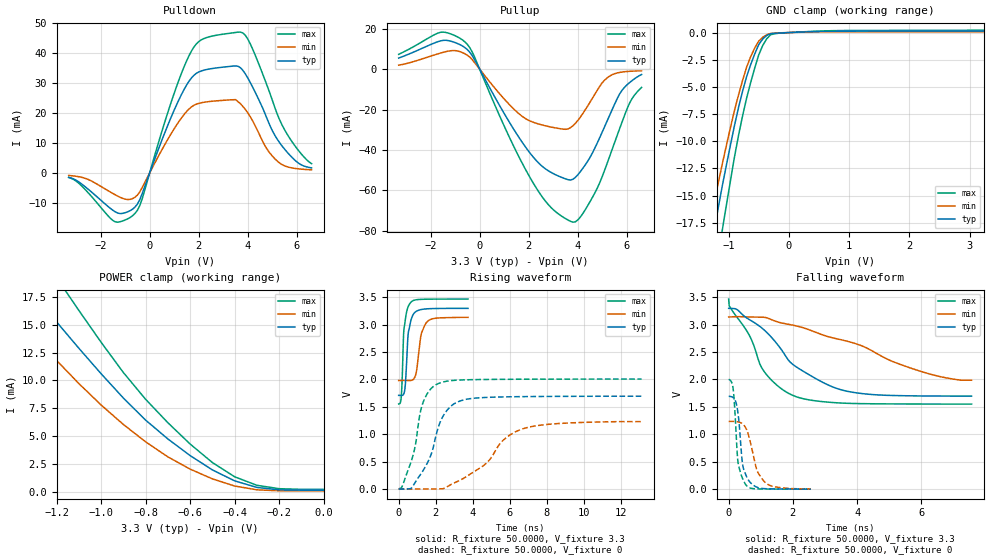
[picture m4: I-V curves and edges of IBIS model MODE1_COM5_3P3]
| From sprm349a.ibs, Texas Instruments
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|MODE4_IND5_3P3BUFFER IN NORMAL MODE WITH INDTEMP AT PLUS OR MINUS 5PERCENT
| VDDS
|COM AND INDE ARE TWO DIFFERENT TEMP MODES.
|COM IS 25,0,105(NOM,STRONG,WEAK)
|IND IS 25,-40,125(NOM,STRONG,WEAK)
|   Model Cell MODE1_COM5_3P3
|MODE1_COM5_3P3
[Model]   MODE1_COM5_3P3
Model_type   I/O
Polarity   Non-Inverting
Enable   Active-Low
Vinl =  0.8V
Vinh =  2V
Cref =  15.0000pF
Rref =  100.0000M
Vref =  0V
Vmeas =  1.65
C_comp   1.505368p   1.470769p   1.543249p
[Model Spec]
Vinl   0.8V   0.8V   0.8V
Vinh   2V   2V   2V
[Temperature Range]   25   105   0
[Voltage Range]   3.3   3.14   3.47
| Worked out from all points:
|   slope of the pulldown table from 0 to 0.495 V, typ, clamps not added: 45.6 ohm
|   slope of the pullup table from 0 to 0.495 V, typ, clamps not added: 44.5 ohm
|   GND clamp passes 1 mA (typ) near -0.49 V on its own axis
|   POWER clamp passes 1 mA (typ) near -0.40 V on its own axis
|   rising waveform, R_fixture 50.0000, V_fixture 3.3: 20-80 % time 216ps typ, 314ps min, 177ps max; typ from 1.71 V to 3.3 V
|   rising waveform, R_fixture 50.0000, V_fixture 0: 20-80 % time 1.12ns typ, 2.25ns min, 778ps max; typ from 0 V to 1.69 V
|   falling waveform, R_fixture 50.0000, V_fixture 3.3: 20-80 % time 1.76ns typ, 3.13ns min, 1.1ns max; typ from 3.3 V to 1.7 V
|   falling waveform, R_fixture 50.0000, V_fixture 0: 20-80 % time 186ps typ, 352ps min, 149ps max; typ from 1.69 V to 0.002 V
[POWER_clamp]
|   voltage   I(typ)   I(min)   I(max)
-3.3V     77.9mA     59.72mA    95.29mA
-1.467V   22.2mA     17.74mA    27.49mA
-1.3V     17.73mA    13.98mA    22.25mA
-1.167V   14.48mA    11.11mA    18.27mA
-1.133V   13.69mA    10.42mA    17.29mA
-900mV    8.425mA    6.05mA     10.72mA
-800mV    6.438mA    4.488mA    8.31mA
-700mV    4.744mA    3.133mA    6.204mA
-500mV    1.961mA    1.156mA    2.623mA
-400mV    976.4uA    512.8uA    1.342mA
-300mV    387.1uA    172.9uA    577.3uA
0V        135.7uA    75.28uA    210.9uA
[Pulldown]
|   voltage   I(typ)   I(min)   I(max)
-3.3V     -1.458mA   -835.8uA   -1.527mA
-1.5V     -12.42mA   -6.829mA   -15.81mA
-700mV    -12.08mA   -8.564mA   -14.28mA
-400mV    -8.847mA   -6.264mA   -10.85mA
900mV     19.04mA    13.41mA    24.14mA
1.7V      31.62mA    21.98mA    40.55mA
2.2V      34.21mA    23.53mA    44.72mA
3.6V      35.53mA    23.76mA    46.9mA
4.1V      30.13mA    18.74mA    43mA
5.2V      11.23mA    3.965mA    19.6mA
6V        3.677mA    1.429mA    8.174mA
6.6V      1.68mA     1.044mA    3.086mA
[Pullup]
|   voltage   I(typ)   I(min)   I(max)
-3.3V     5.462mA    1.977mA    7.321mA
-1.6V     13.96mA    7.929mA    18.2mA
-600mV    10.64mA    7.595mA    13.46mA
-300mV    6.62mA     4.641mA    8.417mA
1.3V      -28.03mA   -18.64mA   -35.96mA
2.2V      -43.74mA   -26.36mA   -56.7mA
2.9V      -51.03mA   -28.63mA   -68.37mA
3.8V      -54.5mA    -28.02mA   -75.74mA
4.4V      -45.62mA   -18.27mA   -67.62mA
5.2V      -25.52mA   -4.294mA   -46.47mA
6.1V      -6.753mA   -1.088mA   -17.05mA
6.6V      -2.667mA   -792.5uA   -9.051mA
[GND_clamp]
|   voltage   I(typ)   I(min)   I(max)
-3.3V     -92.32mA   -71.67mA   -112mA
-1.367V   -22.54mA   -19.08mA   -27.75mA
-1.3V     -20.22mA   -17.26mA   -25.15mA
-1.233V   -18.05mA   -15.48mA   -22.73mA
-1.1V     -13.98mA   -11.97mA   -18.03mA
-900mV    -8.502mA   -7.121mA   -11.38mA
-700mV    -4.041mA   -3.166mA   -6.02mA
-500mV    -1.111mA   -792uA     -2.06mA
-366.7mV  -262.5uA   -199.3uA   -571.7uA
-233.3mV  -71.39uA   -52.59uA   -115.7uA
500mV     96.72uA    58.31uA    132.4uA
3.233V    135.4uA    76.76uA    209.8uA
[Ramp]
| variable   typ   min   max
dV/dt_f  0.9681141/1.780663n   0.7419221/3.397894n   1.159358/1.11711n
dV/dt_r   1.020312/1.126954n   0.7528627/2.318718n   1.207566/0.782362n
R_load = 50
[Rising Waveform]
R_fixture = 50.0000
V_fixture = 3.3
V_fixture_min = 3.14
V_fixture_max = 3.47
|   time   V(typ)   V(min)   V(max)
0s        1.707V     1.98V      1.55V
136ps     1.707V     1.98V      1.664V
264ps     1.728V     1.98V      2.808V
320ps     1.788V     1.98V      2.989V
504ps     2.799V     1.98V      3.319V
592ps     2.965V     1.979V     3.378V
912ps     3.233V     2.077V     3.451V
1.192ns   3.273V     2.783V     3.46V
1.496ns   3.286V     3.037V     3.463V
3.744ns   3.296V     3.132V     3.465V
[Rising Waveform]
R_fixture = 50.0000
V_fixture = 0
V_fixture_min = 0
V_fixture_max = 0
|   time   V(typ)   V(min)   V(max)
0s        45.69uV    22.79uV    74.32uV
192ps     -1.266mV   -593uV     49.17mV
744ps     40.34mV    -4.001mV   575.8mV
1.336ns   345.2mV    -66.73uV   1.594V
1.768ns   645.1mV    -5.992uV   1.838V
2.096ns   1.076V     328.5uV    1.916V
2.6ns     1.432V     35.35mV    1.967V
3.312ns   1.605V     158.7mV    1.988V
6.584ns   1.684V     1.084V     2.002V
13.12ns   1.692V     1.228V     2.005V
[Falling Waveform]
R_fixture = 50.0000
V_fixture = 3.3
V_fixture_min = 3.14
V_fixture_max = 3.47
|   time   V(typ)   V(min)   V(max)
0s        3.297V     3.138V     3.466V
16ps      3.296V     3.14V      3.344V
272ps     3.271V     3.145V     3.125V
648ps     3.09V      3.139V     2.8V
1.096ns   2.907V     3.134V     2.152V
1.976ns   2.285V     2.993V     1.716V
3.104ns   1.898V     2.779V     1.586V
3.848ns   1.768V     2.673V     1.563V
5.952ns   1.7V       2.154V     1.553V
7.568ns   1.696V     1.986V     1.551V
[Falling Waveform]
R_fixture = 50.0000
V_fixture = 0
V_fixture_min = 0
V_fixture_max = 0
|   time   V(typ)   V(min)   V(max)
0s        1.692V     1.235V     2.003V
136ps     1.672V     1.236V     1.843V
184ps     1.64V      1.235V     1.513V
240ps     1.554V     1.232V     921.1mV
304ps     1.319V     1.225V     443.7mV
424ps     498mV      1.194V     206.8mV
544ps     246.9mV    1.104V     73.12mV
888ps     34.08mV    335.1mV    6.047mV
1.16ns    8.843mV    111.1mV    3.033mV
2.56ns    1.745mV    6.39mV     447.4uV
